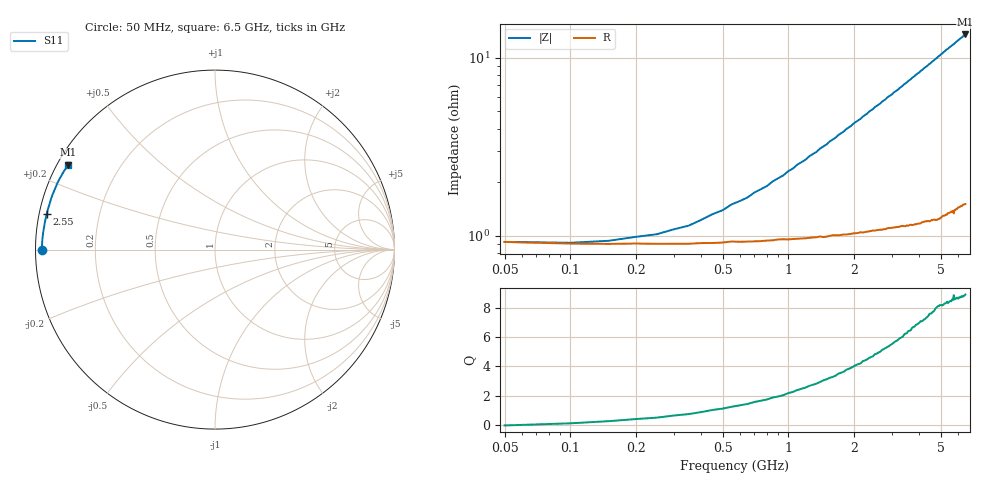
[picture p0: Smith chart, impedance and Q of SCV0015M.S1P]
! Infineon Technologies  Discrete & RF Semiconductors
! BAR63-02L
! Si PIN Diode in TSLP-2
! IF = 15 mA
! S-Parameters:  March  2002
# GHz  S  MA  R  50
!  f  S11
! GHz  MAG  ANG
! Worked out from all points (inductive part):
!   130 points, 50 MHz to 6.5 GHz, reference 50 ohm
!   read as one part to ground: L = 328 pH near 1.45 GHz
!   highest Q = 8.88 at 6.5 GHz (marker M1), where L = 328 pH
!   S11 on the Smith chart (normalised r, x): 50 MHz: 0.02, -0.00; 2.55 GHz: 0.02, +0.11; 6.5 GHz: 0.03, +0.27
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0.05  0.9637 -180.0
0.2  0.9644 179.1
0.35  0.9645 178.4
0.45  0.9642 177.8
0.9  0.9626 175.7
1.25  0.9618 174.0
1.65  0.9606 172.2
1.7  0.9607 171.9
1.8  0.9603 171.5
2  0.9597 170.5
2.15  0.9593 169.9
2.5  0.9585 168.2
2.55  0.9583 168.0
3.3  0.9564 164.6
3.65  0.9558 163.0
3.7  0.956 162.7
3.8  0.9557 162.3
3.85  0.9557 162.0
4.1  0.9547 160.9
4.9  0.9533 157.2
5.3  0.951 155.3
5.65  0.9497 153.8
5.7  0.949 153.5
5.75  0.9506 153.4
5.8  0.9485 153.1
6.05  0.947 152.0
6.1  0.947 151.7
6.5  0.9453 150.0
